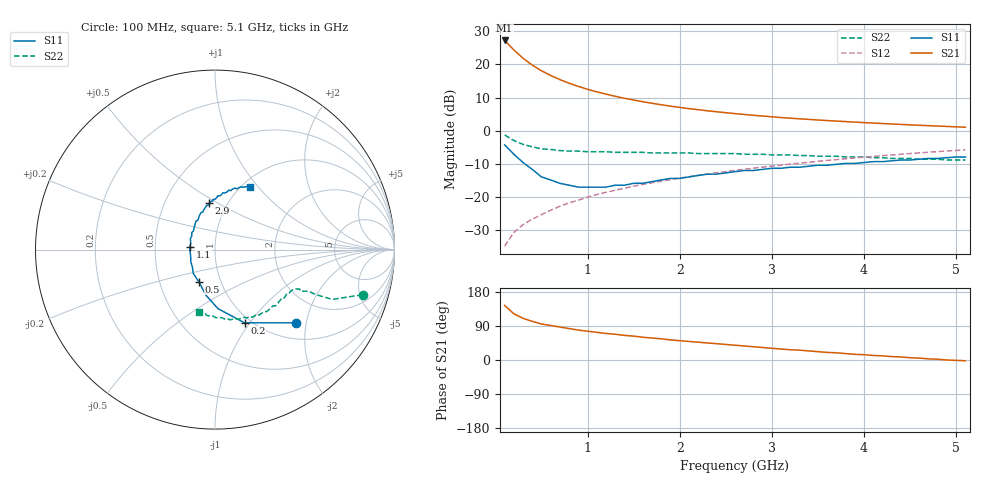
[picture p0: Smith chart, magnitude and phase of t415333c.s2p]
!AT-41533
!S and NOISE PARAMETERS at Vce=2.7V Ic=10mA. LAST UPDATED 01-25-95
# ghz s ma r 50
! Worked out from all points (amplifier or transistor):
!   51 points, 100 MHz to 5.1 GHz, reference 50 ohm
!   highest |S21| = 27.2 dB at 100 MHz (marker M1)
!   |S21| within 3 dB of that: start of sweep to 206 MHz
!   unconditionally stable (mu >= 1): 678.1 MHz to 2.414 GHz
!   at 900 MHz: K = 1.04, MAG = 15.9 dB, |S12| = -21.0 dB
!   at 2.6 GHz: K = 0.98, MSG = 8.6 dB, |S12| = -12.0 dB
!   at 5.1 GHz: K = 0.87, MSG = 3.4 dB, |S12| = -5.8 dB
!   lowest NFmin = 0.80 dB at 100 MHz
!   S11 on the Smith chart (normalised r, x): 100 MHz: 1.35, -1.75; 200 MHz: 0.93, -0.94; 500 MHz: 0.79, -0.29; 1.1 GHz: 0.76, +0.02; 2.9 GHz: 0.82, +0.46; 5.1 GHz: 1.09, +0.91
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0.1  0.61 -42.0  22.99 144.0  0.018 73.0  0.86 -17.0
0.2  0.44 -68.0  16.56 122.0  0.029 67.0  0.71 -23.0
0.3  0.33 -87.0  12.38 110.0  0.038 67.0  0.62 -24.0
0.4  0.26 -101.0  9.756 102.0  0.046 68.0  0.57 -24.0
0.5  0.2 -117.0  8.021 95.0  0.054 68.0  0.53 -26.0
0.6  0.18 -132.0  6.796 91.0  0.063 69.0  0.52 -25.0
0.7  0.16 -142.0  5.897 87.0  0.072 69.0  0.5 -26.0
0.8  0.15 -154.0  5.195 83.0  0.081 70.0  0.49 -27.0
0.9  0.14 -166.0  4.653 79.0  0.089 70.0  0.49 -27.0
1  0.14 -178.0  4.207 76.0  0.099 69.0  0.48 -29.0
1.1  0.14 174.0  3.854 73.0  0.108 69.0  0.48 -30.0
1.2  0.14 165.0  3.556 70.0  0.117 69.0  0.48 -31.0
1.4  0.15 150.0  3.083 65.0  0.135 68.0  0.47 -33.0
1.6  0.16 138.0  2.731 60.0  0.154 66.0  0.47 -36.0
1.8  0.18 128.0  2.457 56.0  0.173 65.0  0.46 -38.0
1.9  0.19 124.0  2.343 53.0  0.182 64.0  0.46 -40.0
2.1  0.2 117.0  2.151 49.0  0.201 63.0  0.46 -43.0
2.6  0.24 103.0  1.806 39.0  0.251 58.0  0.45 -50.0
2.9  0.26 97.0  1.659 33.0  0.281 55.0  0.44 -56.0
3.5  0.3 87.0  1.448 22.0  0.344 49.0  0.41 -67.0
4.3  0.35 74.0  1.259 9.0  0.429 40.0  0.38 -85.0
5.1  0.4 61.0  1.126 -2.0  0.512 29.0  0.36 -104.0
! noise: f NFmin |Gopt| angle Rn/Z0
0.1  0.8  0.21  13  0.14
0.9  1.1  0.14  132  0.11
1.8  1.5  0.38  -142  0.1
2.4  1.7  0.52  -113  0.2
